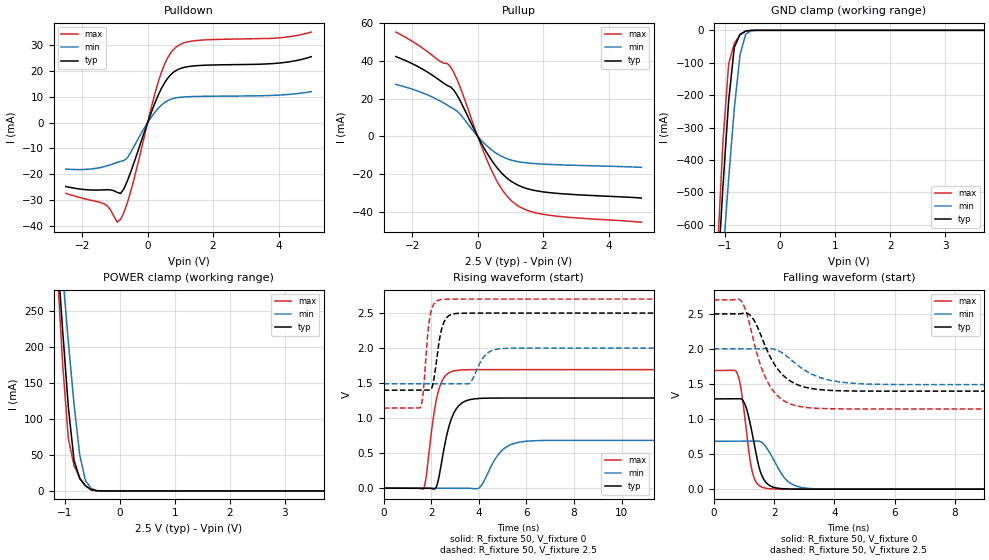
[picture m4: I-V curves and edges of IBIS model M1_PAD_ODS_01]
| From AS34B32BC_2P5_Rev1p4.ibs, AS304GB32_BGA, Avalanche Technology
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[Model] M1_PAD_ODS_01
Model_type I/O
Enable   Active-High
Vinl  =  0.7
Vinh  =  1.8
Vmeas =  1.25
Cref  =  30e-12
| Capacitance   typ   min   max
C_comp   6.259786e-12  5.891456e-12  6.837814e-12
| Variables   typ   min   max
[GND Clamp Reference]   0   0   0
[POWER Clamp Reference]   2.5   2   2.7
[Pulldown Reference]   0   0   0
[Pullup Reference]   2.5   2   2.7
[Temperature Range]   25   125   -40
[Voltage Range]   2.5   2   2.7
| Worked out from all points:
|   slope of the pulldown table from 0 to 0.375 V, typ, clamps not added: 31.1 ohm
|   slope of the pullup table from 0 to 0.375 V, typ, clamps not added: 33 ohm
|   GND clamp passes 1 mA (typ) near -0.56 V on its own axis
|   POWER clamp passes 1 mA (typ) near -0.46 V on its own axis
|   falling waveform, R_fixture 50, V_fixture 0: 20-80 % time 381ps typ, 576ps min, 302ps max; typ from 1.29 V to 0 V
|   falling waveform, R_fixture 50, V_fixture 2.5: 20-80 % time 832ps typ, 1.11ns min, 715ps max; typ from 2.5 V to 1.4 V
|   rising waveform, R_fixture 50, V_fixture 0: 20-80 % time 515ps typ, 728ps min, 426ps max; typ from 0 V to 1.29 V
|   rising waveform, R_fixture 50, V_fixture 2.5: 20-80 % time 302ps typ, 478ps min, 231ps max; typ from 1.4 V to 2.5 V
[GND Clamp]
| Voltage   I(typ)   I(min)   I(max)
-2.5V     -5.188A    -4.586A    -6.153A
-1.138V   -783.9mA   -953.3mA   -701.6mA
-1.034V   -484.9mA   -700.5mA   -347mA
-931mV    -219.3mA   -459.7mA   -104.8mA
-827.6mV  -52.73mA   -241.7mA   -40.47mA
-724.1mV  -12.9mA    -76.61mA   -13.47mA
-620.7mV  -2.491mA   -11.2mA    -1.732mA
-517.2mV  -140.5uA   -1.281mA   -29.11uA
-413.8mV  -3.362uA   -98.11uA   -229.5nA
5V        0A         0A         0A
[POWER Clamp]
| Voltage   I(typ)   I(min)   I(max)
-2.5V     2.044A     1.82A      2.427A
-1.138V   339mA      399.6mA    314.6mA
-1.034V   222.7mA    301.1mA    175.8mA
-931mV    116.3mA    206.8mA    72.64mA
-827.6mV  42.71mA    120.3mA    35.15mA
-724.1mV  16.95mA    49.78mA    18.47mA
-620.7mV  7.083mA    14.35mA    7.103mA
-517.2mV  1.86mA     3.351mA    1.319mA
-413.8mV  190.6uA    480.6uA    44.77uA
-310.3mV  6.062uA    46.87uA    467.4nA
5V        0A         0A         0A
[Pulldown]
| Voltage   I(typ)   I(min)   I(max)
-2.5V     -24.84mA   -18.06mA   -27.47mA
-1.345V   -26.13mA   -17.16mA   -31.47mA
-1.138V   -26.14mA   -16.38mA   -33.83mA
-931mV    -27.08mA   -15.46mA   -38.7mA
-827.6mV  -27.55mA   -15.06mA   -37.59mA
-517.2mV  -19.21mA   -11.59mA   -26.74mA
344.8mV   11.25mA    5.851mA    16.61mA
603.4mV   17.11mA    8.493mA    24.99mA
948.3mV   20.78mA    9.791mA    30.07mA
1.638V    22.25mA    10.22mA    32.08mA
3.99V     23.14mA    10.7mA     32.95mA
5V        25.64mA    12.06mA    35.21mA
[Pullup]
| Voltage   I(typ)   I(min)   I(max)
-2.5V     42.42mA    27.62mA    55.43mA
-1.552V   34.36mA    22.2mA     45.21mA
-827.6mV  26.25mA    15.56mA    36.93mA
-724.1mV  24.46mA    14.55mA    33.66mA
-517.2mV  18.3mA     11.42mA    25.3mA
86.21mV   -2.826mA   -1.658mA   -4mA
431mV     -12.85mA   -7.255mA   -18.38mA
775.9mV   -20.27mA   -10.97mA   -29.06mA
1.121V    -24.9mA    -13.01mA   -35.54mA
1.552V    -27.96mA   -14.16mA   -39.52mA
2.069V    -29.63mA   -14.78mA   -41.6mA
5V        -32.74mA   -16.44mA   -45.58mA
[Ramp]
dV/dt_r   0.772527/0.51492n  0.409943/0.728462n  1.01555/0.426032n
dV/dt_f   0.661206/0.831778n  0.305568/1.10889n  0.934102/0.714898n
R_load = 50
[Falling Waveform]
R_fixture = 50
V_fixture = 0
V_fixture_min = 0
V_fixture_max = 0
| Time   V(typ)   V(min)   V(max)
0s        1.288V     683.2mV    1.693V
776.4ps   1.288V     683.7mV    1.654V
905ps     1.289V     683.8mV    1.427V
1.023ns   1.221V     683.9mV    1.05V
1.27ns    800.9mV    684.1mV    259.5mV
1.497ns   318.7mV    685.9mV    54.9mV
1.694ns   116.3mV    623.8mV    15.38mV
2.424ns   3.235mV    124.1mV    741.7uV
3.248ns   251.5uV    7.781mV    710.3uV
21.88ns   -42.9nV    426.2nV    30.53nV
[Falling Waveform]
R_fixture = 50
V_fixture = 2.5
V_fixture_min = 2
V_fixture_max = 2.7
| Time   V(typ)   V(min)   V(max)
0s        2.5V       2V         2.7V
907.7ps   2.504V     2.001V     2.686V
1.265ns   2.455V     2.001V     2.216V
1.537ns   2.221V     2.003V     1.787V
1.834ns   1.919V     2.008V     1.49V
2.242ns   1.65V      1.952V     1.285V
2.817ns   1.483V     1.757V     1.182V
3.595ns   1.417V     1.582V     1.15V
4.944ns   1.399V     1.502V     1.144V
21.88ns   1.398V     1.491V     1.143V
[Rising Waveform]
R_fixture = 50
V_fixture = 0
V_fixture_min = 0
V_fixture_max = 0
| Time   V(typ)   V(min)   V(max)
0s        7.49nV     250.4nV    6.615nV
1.671ns   -818.4uV   -176.7uV   -5.916mV
2.162ns   -7.688mV   -228.7uV   1.168V
2.301ns   122.1mV    -243.4uV   1.387V
2.69ns    811.1mV    -284.5uV   1.635V
2.96ns    1.08V      -313.1uV   1.675V
3.991ns   1.281V     -310.2uV   1.692V
4.949ns   1.287V     531.8mV    1.693V
5.957ns   1.287V     668.9mV    1.693V
21.88ns   1.288V     683.2mV    1.693V
[Rising Waveform]
R_fixture = 50
V_fixture = 2.5
V_fixture_min = 2
V_fixture_max = 2.7
| Time   V(typ)   V(min)   V(max)
0s        1.398V     1.491V     1.143V
1.551ns   1.399V     1.491V     1.154V
1.664ns   1.399V     1.491V     1.371V
1.942ns   1.398V     1.491V     2.444V
2.411ns   2.236V     1.491V     2.692V
2.735ns   2.461V     1.492V     2.699V
3.59ns    2.5V       1.494V     2.7V
4.277ns   2.5V       1.902V     2.7V
4.988ns   2.5V       1.994V     2.7V
21.88ns   2.5V       2V         2.7V
